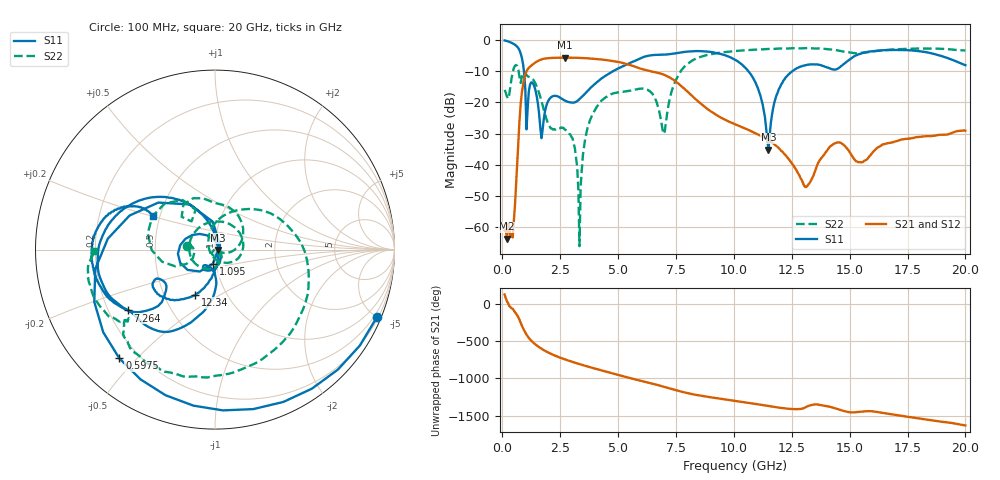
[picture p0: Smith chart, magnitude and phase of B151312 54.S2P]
!  2-Port S-parameters saved by WinCal
! VAR MeasName=S-Parameters (CALIBRATED_DATA) read from VNA (N5244A)
! VAR MeasDate=12/8/2015 5:48:00 PM
! VAR NAME=B151312 54
! VAR FILENAME=B151312 54.S2P
! VAR DATE=12/8/2015 5:48:00 PM
! VAR PHYS_PORTS=1,2
# Hz S DB R 50
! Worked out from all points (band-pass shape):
!   401 points, 100 MHz to 20 GHz, reference 50 ohm
!   highest |S21| = -5.70 dB at 2.687 GHz (marker M1); lowest = -63.7 dB at 199.5 MHz (marker M2)
!   |S21| within 3 dB of the highest: 1.181 GHz to 5.771 GHz (4.59 GHz wide, 132 % of centre)
!   lowest |S11| = -35.2 dB at 11.49 GHz (marker M3), VSWR 1.04, Z = 51.8 - j0.168 ohm
!   |S11| at or under -10 dB: 933.2 MHz to 4.79 GHz (3.857 GHz wide, 135 % of centre); 10.62 GHz to 12.53 GHz (1.907 GHz wide, 16.5 % of centre)
!   |S22| runs from -66.0 to -2.6 dB; largest |S21 - S12| = 0.0018
!   S11 on the Smith chart (normalised r, x): 100 MHz: 0.29, -4.99; 597.5 MHz: 0.13, -0.45; 1.095 GHz: 0.96, -0.15; 7.264 GHz: 0.28, -0.29; 12.34 GHz: 0.71, -0.39; 20 GHz: 0.46, +0.20
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1e8  -0.20 -22.6  -61.00 123.1  -61.73 123.2  -16.02 172.6
1.995e8  -0.38 -44.4  -63.69 34.3  -64.64 38.6  -18.10 174.0
4.4825e8  -1.13 -97.9  -63.26 -67.4  -62.95 -66.6  -10.40 -167.0
5.975e8  -1.86 -131.3  -45.98 -133.5  -45.93 -134.6  -8.06 152.1
8.4625e8  -5.81 158.2  -16.83 65.3  -16.83 65.3  -11.69 135.5
1.095e9  -21.99 -98.5  -9.42 -77.3  -9.42 -77.4  -11.67 91.4
1.44325e9  -16.48 147.2  -7.19 171.8  -7.19 171.8  -14.14 36.9
1.84125e9  -22.97 -66.8  -5.99 89.4  -5.99 89.4  -23.65 -16.7
2.687e9  -19.37 -125.3  -5.70 -24.3  -5.70 -24.3  -28.61 -83.7
3.43325e9  -18.26 -94.0  -5.82 -98.6  -5.81 -98.6  -41.49 -5.2
3.682e9  -16.37 -88.7  -5.91 -121.2  -5.91 -121.2  -28.13 -34.6
4.32875e9  -12.13 -91.1  -6.33 -177.3  -6.33 -177.4  -19.17 -102.6
5.32375e9  -8.05 -105.4  -7.64 99.1  -7.61 99.0  -16.53 135.5
6.7665e9  -4.79 -137.3  -10.65 -14.4  -10.65 -14.5  -22.51 -66.4
7.264e9  -4.54 -145.1  -12.20 -58.6  -12.18 -58.8  -17.85 96.1
8.458e9  -3.59 -169.8  -19.70 -146.7  -19.70 -147.2  -5.73 -7.0
1.005e10  -6.34 143.9  -27.04 138.9  -27.04 138.6  -3.60 -65.2
1.149275e10  -35.15 -5.3  -32.07 69.5  -32.11 69.5  -2.92 -94.8
1.23385e10  -11.20 -113.6  -37.88 32.5  -37.85 32.0  -2.76 -108.9
1.338325e10  -7.84 -144.7  -44.23 84.0  -44.16 83.6  -2.74 -124.0
1.67165e10  -3.29 -171.2  -33.00 -38.9  -32.96 -39.6  -3.14 -147.5
2e10  -8.12 151.7  -29.07 168.2  -29.16 167.7  -3.42 -179.2
